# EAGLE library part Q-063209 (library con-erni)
Male Connector SMC-Q 26 contacts Standard Assembly Height Source: http://www.erni.com/DB/PDF-Drawing/SMC/063209.pdf
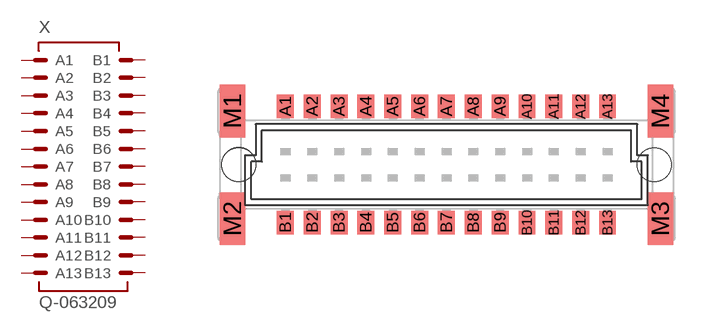
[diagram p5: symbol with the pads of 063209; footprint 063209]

Designator prefix X

## Q-063209 (OC_FARNELL: unknown; OC_NEWARK: unknown)  [063209]
A1  A1  pas
A2  A2  pas
A3  A3  pas
A4  A4  pas
A5  A5  pas
A6  A6  pas
A7  A7  pas
A8  A8  pas
A9  A9  pas
A10  A10  pas
A11  A11  pas
A12  A12  pas
A13  A13  pas
B1  B1  pas
B2  B2  pas
B3  B3  pas
B4  B4  pas
B5  B5  pas
B6  B6  pas
B7  B7  pas
B8  B8  pas
B9  B9  pas
B10  B10  pas
B11  B11  pas
B12  B12  pas
B13  B13  pas

## Footprint 063209 (pad centres in mm)
Male Connector SMC-Q 26 contacts Standard Assembly Height Source: http://www.erni.com/DB/PDF-Drawing/SMC/063209.pdf
smd 0.8 x 1.1: A1 -7.62,2.765; A2 -6.35,2.765; A3 -5.08,2.765; A4 -3.81,2.765; A5 -2.54,2.765; A6 -1.27,2.765; A7 0,2.765; A8 1.27,2.765; A9 2.54,2.765; A10 3.81,2.765; A11 5.08,2.765; A12 6.35,2.765; A13 7.62,2.765; B1 -7.62,-2.74; B2 -6.35,-2.74; B3 -5.08,-2.74; B4 -3.81,-2.74; B5 -2.54,-2.74; B6 -1.27,-2.74; B7 0,-2.74; B8 1.27,-2.74; B9 2.54,-2.74; B10 3.81,-2.74; B11 5.08,-2.74; B12 6.35,-2.74; B13 7.62,-2.74
smd 1.2 x 2.5: M1 -10.125,2.55; M2 -10.125,-2.55; M3 10.125,-2.55; M4 10.125,2.55
hole 1.6 at -9.83,0
hole 1.6 at 9.83,0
